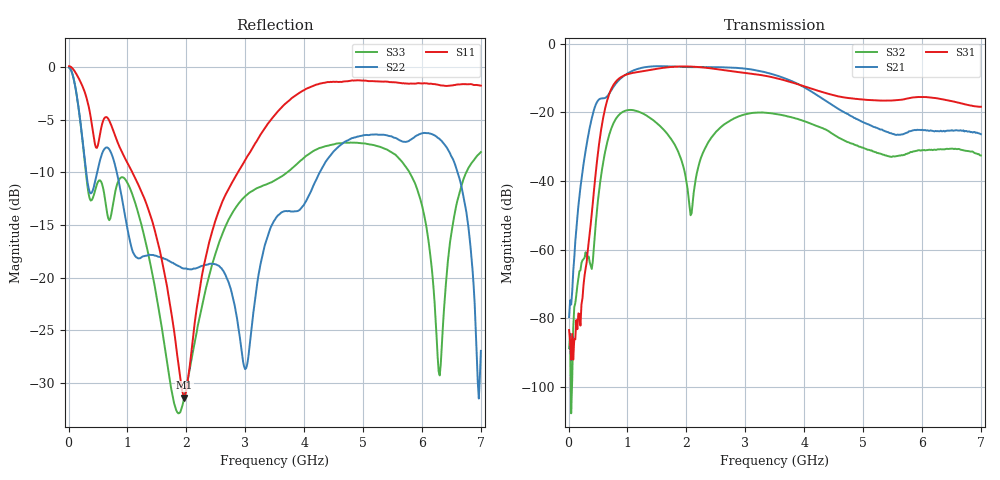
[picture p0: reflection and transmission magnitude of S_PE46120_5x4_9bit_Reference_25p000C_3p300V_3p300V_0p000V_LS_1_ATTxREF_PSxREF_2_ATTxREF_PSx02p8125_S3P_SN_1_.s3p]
! Device ID: PE46120_5x4_9bit_Reference
! Device ID: PE46120_5x4_9bit_Reference
! File Path: z:\PE46120_5x4_9bit_Reference\MPAC_Yi\new_12port\25p000C\3p300\LS_1_ATTxREF_PSxREF_2_ATTxREF_PSx02p8125\PE46120_5x4_9bit_Reference_25p000C_3p300V_3p300V_0p000V_LS_1_ATTxREF_PSxREF_2_ATTxREF_PSx02p8125_S3P_SN_1_.s3p
! Serial: 1
! Lot:
! Temp: 25.000C
! VDD: 3.300
! VSS: 0.000
! Control_Hi: 3.300
! Control_Lo: 0.000
! Logic State: LS_1_ATTxREF_PSxREF_2_ATTxREF_PSx02p8125
! Port 1: RFin
! Port 2: RFout1
! Port 3: RFout2
! ThroughPath:1-3
! IDD: -0.0005451218
! ISS: 0
! Comment:
#  Hz  S  RI  R  50
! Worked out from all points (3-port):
!   401 points, 10 MHz to 7 GHz, reference 50 ohm
!   strongest paths, dB at 10 MHz, 1.758 GHz, 3.505 GHz, 5.253 GHz, 7 GHz:
!     S31: -83.4, -6.7, -9.9, -16.5, -18.4
!     S21: -79.6, -6.6, -9.1, -24.7, -26.4
!     S32: -88.7, -28.2, -20.4, -31.8, -32.6
!   lowest |S11| = -31.4 dB at 1.967 GHz (marker M1), VSWR 1.06, Z = 52.6 + j1.03 ohm
!   |S11| at or under -10 dB: 1.082 GHz to 2.876 GHz (1.794 GHz wide, 90.6 % of centre)
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1e7  1.001 -0.1152  0.000113 6.72e-06  7.81e-05 -1.79e-05
     8.99e-05 5.27e-05  0.9873 -0.0966  -8.26e-06 2.82e-06
     5.07e-05 4.42e-05  3.64e-05 3.61e-06  0.9874 -0.0963
2.37175e8  -0.4718 -0.6575  -0.0128 -0.00483  0.000101 0.000211
           -0.0128 -0.00496  -0.2855 -0.3506  -0.000325 0.000551
           2.46e-05 0.000195  -0.000311 0.000626  -0.2833 -0.3444
4.6435e8  -0.408 -0.0737  -0.0555 0.1162  0.0133 0.00298
          -0.0563 0.1179  0.1376 0.2645  -0.00176 0.00173
          0.0134 0.00308  -0.00188 0.00167  0.1671 0.2092
9.187e8  -0.2986 0.248  0.3248 -0.0225  -0.1373 0.302
         0.3291 -0.023  -0.0355 -0.2259  -0.0692 0.0729
         -0.1391 0.3061  -0.0699 0.0736  0.1117 -0.2778
1.9672e9  0.0251 0.00981  -0.3774 0.2491  -0.2817 -0.3651
          -0.3818 0.2524  -0.0933 0.059  0.00132 0.0139
          -0.2855 -0.3691  0.00136 0.014  -0.025 0.011
2.806e9  -0.0733 -0.2829  0.4325 0.0922  -0.0697 0.3825
         0.4385 0.0928  0.0716 -0.0286  0.0171 0.0783
         -0.0699 0.3875  0.0177 0.0794  0.1187 0.1708
3.505e9  -0.4378 -0.4006  -0.0944 -0.3328  0.3132 0.0231
         -0.0956 -0.3373  0.0633 0.1776  0.00234 -0.0943
         0.3174 0.0233  0.00217 -0.0954  0.151 -0.2471
5.619475e9  -0.6234 0.5619  0.0442 0.0144  -0.1331 0.0685
            0.0447 0.0151  0.3421 0.2903  0.012 -0.0197
            -0.1348 0.0696  0.0124 -0.0199  0.3531 0.0945
6.301e9  -0.3563 0.7374  0.0371 -0.0371  0.0404 0.1502
         0.0374 -0.0375  0.4345 -0.1323  -0.0264 0.00779
         0.0413 0.1516  -0.028 0.00744  0.0306 0.0156
7e9  -0.1112 0.8073  -0.0295 -0.0374  0.116 0.0249
     -0.0297 -0.0378  -0.0348 0.0286  0.0232 0.00175
     0.118 0.0247  0.0235 0.00184  0.2001 0.3398
